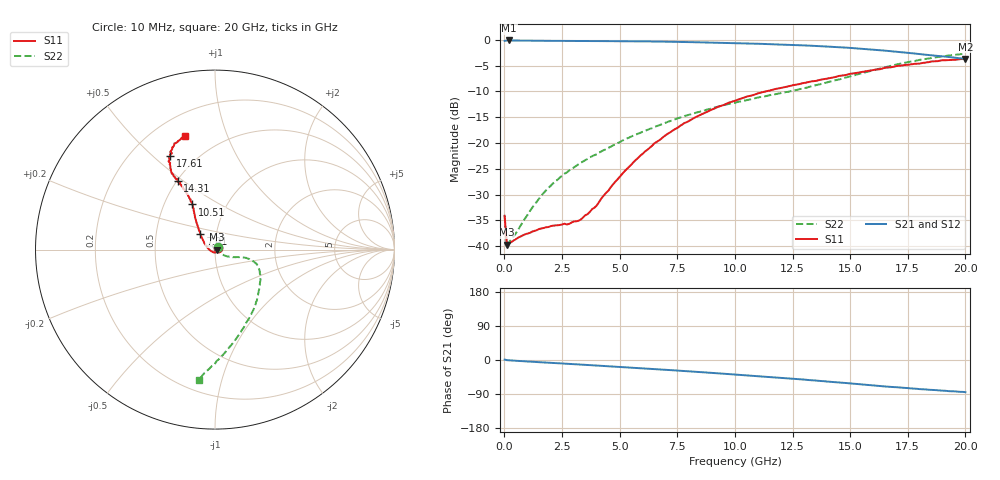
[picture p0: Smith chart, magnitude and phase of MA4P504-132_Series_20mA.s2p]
! AWR Design Environment (9226) Thu Aug 19 02:45:16 2021
! Document = '20mA'
! nPorts: 2, nXvals: 201
# GHz S DB R 50
!Freq DBS11 AngS11 DBS21 AngS21 DBS12 AngS12 DBS22 AngS22
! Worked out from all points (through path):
!   201 points, 10 MHz to 20 GHz, reference 50 ohm
!   highest |S21| = -0.14 dB at 210 MHz (marker M1); lowest = -3.7 dB at 20 GHz (marker M2)
!   group delay of S21, straight-line fit = 12 ps
!   lowest |S11| = -39.7 dB at 110 MHz (marker M3), VSWR 1.02, Z = 51 + j0.00125 ohm
!   |S11| at or under -10 dB: start of sweep to 11.34 GHz
!   |S22| runs from -40.0 to -2.7 dB; largest |S21 - S12| = 0.031
!   S11 on the Smith chart (normalised r, x): 10 MHz: 1.04, +0.01; 7.01 GHz: 0.84, +0.15; 10.51 GHz: 0.69, +0.38; 14.31 GHz: 0.51, +0.47; 17.61 GHz: 0.36, +0.57; 20 GHz: 0.33, +0.72
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0.01  -34.09 21.2  -0.22 1.2  -0.16 0.4  -34.01 38.1
0.11  -39.71 0.1  -0.14 -0.4  -0.13 -0.5  -39.97 -0.0
0.21  -39.40 -1.3  -0.14 -0.9  -0.13 -0.9  -39.20 -0.8
0.91  -37.66 -20.7  -0.17 -3.6  -0.16 -3.5  -34.54 -18.0
1.71  -36.45 -49.7  -0.20 -6.4  -0.19 -6.3  -29.64 -28.9
2.71  -35.78 -95.9  -0.23 -9.9  -0.22 -9.6  -25.69 -32.4
3.41  -34.44 -134.9  -0.24 -12.4  -0.24 -12.0  -23.58 -31.1
4.01  -32.08 -164.9  -0.25 -14.6  -0.25 -14.1  -22.18 -28.7
5.21  -25.48 157.7  -0.29 -19.0  -0.28 -18.3  -19.37 -23.3
5.91  -22.40 145.1  -0.31 -21.6  -0.32 -20.9  -17.97 -19.0
6.71  -19.49 135.9  -0.35 -24.7  -0.35 -24.0  -16.57 -16.7
7.01  -18.44 133.3  -0.37 -25.9  -0.37 -25.1  -16.03 -16.1
8.31  -14.96 124.8  -0.48 -31.1  -0.48 -30.2  -14.14 -15.3
10.01  -11.80 117.5  -0.66 -38.4  -0.65 -36.9  -12.19 -19.2
10.51  -11.02 116.7  -0.72 -40.5  -0.70 -39.0  -11.70 -21.9
12.11  -9.22 116.7  -0.95 -47.4  -0.89 -45.9  -10.24 -34.9
13.41  -8.02 117.8  -1.18 -53.7  -1.09 -52.2  -8.92 -48.6
14.31  -7.26 118.7  -1.40 -58.1  -1.28 -56.7  -7.89 -58.6
16.71  -5.37 117.8  -2.19 -70.7  -2.08 -69.4  -5.11 -82.1
17.61  -4.78 115.6  -2.58 -74.9  -2.49 -74.0  -4.25 -88.2
19.01  -3.97 111.0  -3.20 -80.7  -3.23 -80.5  -3.23 -94.8
20  -3.70 104.8  -3.71 -84.9  -3.82 -84.3  -2.70 -97.1
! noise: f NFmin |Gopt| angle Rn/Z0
0.01  0  1  0  2e-20
2.21  0  1  0  2e-20
4.41  0  1  0  2e-20
6.61  0  1  0  2e-20
8.81  0  1  0  2e-20
11.11  0  1  0  2e-20
13.31  0  1  0  2e-20
15.51  0  1  0  2e-20
17.71  0  1  0  2e-20
20  0  1  0  2e-20
